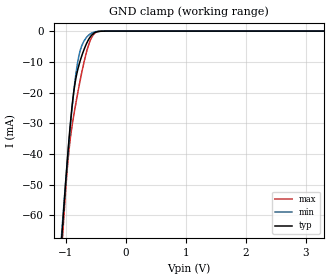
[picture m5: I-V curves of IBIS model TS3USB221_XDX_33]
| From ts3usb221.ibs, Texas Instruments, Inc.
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[Model]   TS3USB221_XDX_33
Model_type  Terminator
| variable   typ   min   max
C_comp   2.10pF   1.81pF   2.36pF
| C_tri-state   2.10pF   1.81pF   2.36pF
[Temperature Range]   40   100   -40
| Ambient temperature   25   85   -40
[Voltage range]   3.3   3   3.6
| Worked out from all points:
|   GND clamp passes 1 mA (typ) near -0.55 V on its own axis
[GND Clamp]
| TS3USB221_XDX_33
|   Voltage   I(typ)   I(min)   I(max)
-3.3V     -844.8mA   -772.7mA   -915.4mA
-1.065V   -66.5mA    -64.75mA   -70.41mA
-1.05V    -62.23mA   -60.9mA    -65.72mA
-975mV    -42.04mA   -42.43mA   -44.75mA
-920mV    -29.22mA   -30.05mA   -34.18mA
-870mV    -20.14mA   -20.16mA   -27.72mA
-820mV    -14.17mA   -12.29mA   -22.14mA
-725mV    -7.533mA   -4.357mA   -12.61mA
-630mV    -3.083mA   -1.519mA   -5.112mA
-565mV    -1.227mA   -594.1uA   -1.898mA
-330mV    -4.709uA   -3.685uA   -2.048uA
3.3V      756.7pA    1.28nA     73.97pA
